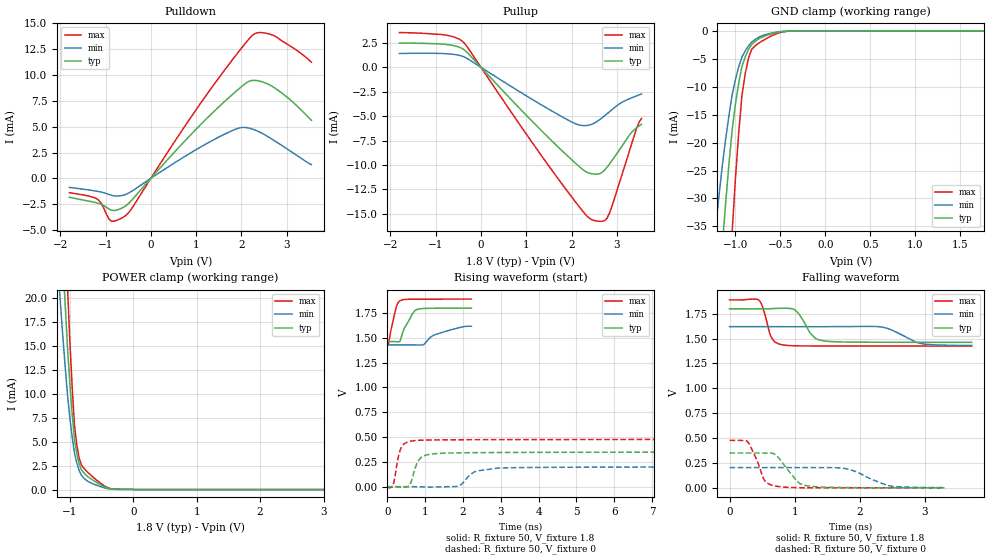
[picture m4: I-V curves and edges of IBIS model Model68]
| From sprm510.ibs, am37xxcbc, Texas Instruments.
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| Model based on original model for BQUSIM1833DVHYPBFZLP18NOPM_SSCHH
|   Sub model 18NOPM_SSCHH_PD1_1P8
[model]   Model68
|[Input Load]   PD
|[Output Drive]
|Voltage   1.8V
|Mode   I/O
Model_type   I/O
Polarity   Non-Inverting
Enable   Active-Low
Vinl =  0.54
Vinh =  1.26
Cref =  15pF
Rref =  100.0000M
Vref =  0V
Vmeas =  0.9
C_comp   1.861602p   1.830694p   1.903969p
[Model Spec]
Vinl   0.54   0.486   0.567
Vinh   1.26   1.134   1.323
[Temperature Range]   25   125   -40
[Voltage Range]   1.8   1.62   1.89
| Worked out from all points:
|   slope of the pulldown table from 0 to 0.27 V, typ, clamps not added: 203 ohm
|   slope of the pullup table from 0 to 0.27 V, typ, clamps not added: 200 ohm
|   GND clamp passes 1 mA (typ) near -0.69 V on its own axis
|   POWER clamp passes 1 mA (typ) near -0.64 V on its own axis
|   rising waveform, R_fixture 50, V_fixture 1.8: 20-80 % time 262ps typ, 624ps min, 160ps max; typ from 1.46 V to 1.8 V
|   rising waveform, R_fixture 50, V_fixture 0: 20-80 % time 209ps typ, 405ps min, 153ps max; typ from 0 V to 0.349 V
|   falling waveform, R_fixture 50, V_fixture 1.8: 20-80 % time 196ps typ, 345ps min, 120ps max; typ from 1.8 V to 1.46 V
|   falling waveform, R_fixture 50, V_fixture 0: 20-80 % time 257ps typ, 409ps min, 175ps max; typ from 0.351 V to 0.001 V
[POWER_clamp]
-1.8V     131.5mA    94.5mA     182.1mA
-1.182V   33.76mA    22.72mA    48.24mA
-1.145V   28.61mA    19.12mA    40.98mA
-1.109V   23.76mA    15.82mA    34.05mA
-1.073V   19.13mA    12.72mA    27.38mA
-1.036V   14.74mA    9.82mA     20.97mA
-963.6mV  7.892mA    5.466mA    10.69mA
-927.3mV  5.251mA    3.798mA    6.697mA
-854.5mV  2.727mA    2.027mA    3.309mA
-709.1mV  1.314mA    835.8uA    1.744mA
-309.1mV  43.86uA    30.44uA    55.56uA
3.6V      0A         0A         0A
[Pulldown]
-1.8V     -1.828mA   -873.3uA   -1.385mA
-1.2V     -2.358mA   -1.237mA   -1.965mA
-1.091V   -2.51mA    -1.332mA   -2.432mA
-927.3mV  -2.959mA   -1.552mA   -3.908mA
-872.7mV  -3.077mA   -1.631mA   -4.142mA
-545.5mV  -2.629mA   -1.532mA   -3.555mA
709.1mV   3.423mA    2.009mA    4.77mA
1.582V    7.249mA    4.174mA    10.2mA
1.964V    8.732mA    4.891mA    12.39mA
2.291V    9.481mA    4.693mA    13.99mA
2.727V    8.774mA    3.647mA    13.79mA
3.545V    5.62mA     1.322mA    11.24mA
[Pullup]
-1.8V     2.468mA    1.407mA    3.554mA
-818.2mV  2.361mA    1.402mA    3.325mA
-381.8mV  1.828mA    1.082mA    2.546mA
1.964V    -9.297mA   -5.505mA   -13.03mA
2.236V    -10.43mA   -5.962mA   -14.67mA
2.455V    -10.91mA   -5.824mA   -15.62mA
2.618V    -10.9mA    -5.37mA    -15.77mA
2.727V    -10.54mA   -4.977mA   -15.71mA
2.836V    -9.913mA   -4.562mA   -14.96mA
3.273V    -6.975mA   -3.239mA   -8.659mA
3.436V    -6.195mA   -2.926mA   -6.256mA
3.545V    -5.839mA   -2.725mA   -5.231mA
[GND_clamp]
-1.8V     -212.9mA   -139.2mA   -381.7mA
-1.218V   -55.61mA   -34.83mA   -107mA
-1.145V   -38.49mA   -24.06mA   -75.74mA
-1.109V   -30.9mA    -19.42mA   -61.46mA
-1.036V   -17.71mA   -11.44mA   -36.01mA
-963.6mV  -9.341mA   -6.449mA   -18.33mA
-927.3mV  -6.372mA   -4.665mA   -11.56mA
-854.5mV  -3.333mA   -2.674mA   -4.883mA
-818.2mV  -2.379mA   -1.984mA   -3.257mA
-745.5mV  -1.448mA   -1.168mA   -2.226mA
-381.8mV  -14.84uA   -16.32uA   -25.73uA
1.764V    22.31uA    13.55uA    30.99uA
[Ramp]
dV/dt_f  0.2058685/0.1864283n  0.1163973/0.3563036n  0.2827081/0.1205513n
dV/dt_r  0.2155895/0.209332n   0.1252084/0.3882558n  0.2935097/0.1552802n
R_load = 50
[Rising Waveform]
R_fixture = 50
V_fixture = 1.8
V_fixture_min = 1.62
V_fixture_max = 1.89
0s        1.461V     1.428V     1.421V
44ps      1.461V     1.428V     1.46V
110ps     1.461V     1.428V     1.601V
242ps     1.46V      1.428V     1.817V
352ps     1.481V     1.428V     1.875V
462ps     1.604V     1.428V     1.885V
770ps     1.782V     1.427V     1.888V
968ps     1.794V     1.432V     1.889V
1.298ns   1.797V     1.535V     1.889V
2.222ns   1.798V     1.616V     1.889V
[Rising Waveform]
R_fixture = 50
V_fixture = 0
V_fixture_min = 0
V_fixture_max = 0
0s        -16.19uV   -107.7uV   -3.942mV
154ps     645.3uV    57.97uV    19.14mV
374ps     -8.239mV   -17.95uV   398.3mV
572ps     7.426mV    282.1uV    453.7mV
770ps     223.1mV    -424.1uV   465.6mV
1.056ns   321.4mV    -4.963mV   470mV
1.892ns   340.8mV    5.976mV    472.6mV
2.354ns   342.7mV    157.5mV    473.2mV
2.926ns   344.1mV    187.4mV    473.8mV
16.21ns   348.8mV    200.4mV    476.4mV
[Falling Waveform]
R_fixture = 50
V_fixture = 1.8
V_fixture_min = 1.62
V_fixture_max = 1.89
0s        1.799V     1.619V     1.889V
462ps     1.799V     1.619V     1.879V
638ps     1.801V     1.619V     1.517V
792ps     1.804V     1.619V     1.439V
1.012ns   1.784V     1.619V     1.427V
1.232ns   1.56V      1.619V     1.426V
1.386ns   1.484V     1.619V     1.426V
2.354ns   1.463V     1.615V     1.425V
2.948ns   1.462V     1.449V     1.425V
3.718ns   1.462V     1.431V     1.425V
[Falling Waveform]
R_fixture = 50
V_fixture = 0
V_fixture_min = 0
V_fixture_max = 0
0s        350.6mV    203.6mV    477.2mV
286ps     350.5mV    203.7mV    457.1mV
418ps     350.3mV    203.7mV    279.5mV
528ps     349.9mV    203.6mV    84.82mV
682ps     342.5mV    203.6mV    21.5mV
1.012ns   86.71mV    203.5mV    2.525mV
1.144ns   26.07mV    203.5mV    1.238mV
1.804ns   3.095mV    190.5mV    221.3uV
2.486ns   1.294mV    17.03mV    123.7uV
3.3ns     741.1uV    3.326mV    83.19uV
